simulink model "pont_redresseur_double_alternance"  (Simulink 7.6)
settings: Solver=ode15s  StartTime=0.0  StopTime=0.05  RelTol=1e-3
StopFcn:
  | close all
  | load signaux.mat
  | plot(x(1,:),x(2,:),x(1,:),x(3,:))
  | title('Sinusoide d''entrée et après redressement')
  | grid
  | xlabel('temps')
libraries: fl_lib x13, nesl_utility x3

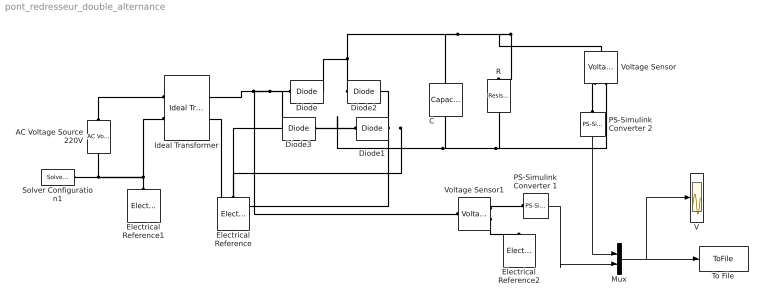
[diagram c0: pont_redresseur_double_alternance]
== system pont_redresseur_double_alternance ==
  AC Voltage Source 220V : fl_lib/Electrical/Electrical Sources/AC Voltage Source  DialogController=NetworkEngine.DynNeDlgSource  SystemSampleTime=-1  amp=220 V  shift=0 rad  omega=60 Hz  i_Log=off  v_Log=off  LocalVarNames=|i|v  LocalVarDescs=|i|v  LocalVarLogging=[0 0]
  C : fl_lib/Electrical/Electrical Elements/Capacitor  DialogController=NetworkEngine.DynNeDlgSource  SystemSampleTime=-1  c=1e-03 F  v0=0 V  r=1e-06 Ohm  g=0 1/Ohm  i_Log=off  v_Log=off  vc_Log=off  LocalVarNames=|i|v|vc  LocalVarDescs=|i|v|Internal variable for voltage across capacitor term  LocalVarLogging=[0 0 0]
  Diode{,1..3} (4 alike) : fl_lib/Electrical/Electrical Elements/Diode  DialogController=NetworkEngine.DynNeDlgSource  SystemSampleTime=-1  Vf=0.6 V  Ron=0.3 Ohm  Goff=1e-08 1/Ohm  i_Log=off  v_Log=off  LocalVarNames=|i|v  LocalVarDescs=|i|v  LocalVarLogging=[0 0]
  Electrical Reference : fl_lib/Electrical/Electrical Elements/Electrical Reference  DialogController=NetworkEngine.DynNeDlgSource  SystemSampleTime=-1  i_Log=off  LocalVarNames=|i  LocalVarDescs=|i  LocalVarLogging=0
  Electrical Reference1 : fl_lib/Electrical/Electrical Elements/Electrical Reference  DialogController=NetworkEngine.DynNeDlgSource  SystemSampleTime=-1  i_Log=off  LocalVarNames=|i  LocalVarDescs=|i  LocalVarLogging=0
  Electrical Reference2 : fl_lib/Electrical/Electrical Elements/Electrical Reference  DialogController=NetworkEngine.DynNeDlgSource  SystemSampleTime=-1  i_Log=off  LocalVarNames=|i  LocalVarDescs=|i  LocalVarLogging=0
  Ideal Transformer : fl_lib/Electrical/Electrical Elements/Ideal Transformer  DialogController=NetworkEngine.DynNeDlgSource  SystemSampleTime=-1  n=18  i1_Log=off  v1_Log=off  i2_Log=off  v2_Log=off  LocalVarNames=|i1|v1|i2|v2  LocalVarDescs=|i1|v1|i2|v2  LocalVarLogging=[0 0 0 0]
  Mux : Mux  Inputs=2
  PS-Simulink Converter 1 : nesl_utility/PS-Simulink Converter  DialogController=NetworkEngine.DynNeUtilDlgSource  SystemSampleTime=-1  PhysicalDomain=network_engine_domain  LeftPortType=input  RightPortType=output  SubClassName=ps_output  Unit=1  AffineConversion=off
  PS-Simulink Converter 2 : nesl_utility/PS-Simulink Converter  DialogController=NetworkEngine.DynNeUtilDlgSource  SystemSampleTime=-1  PhysicalDomain=network_engine_domain  LeftPortType=input  RightPortType=output  SubClassName=ps_output  Unit=1  AffineConversion=off
  R : fl_lib/Electrical/Electrical Elements/Resistor  Tag=Factory Generic  DialogController=NetworkEngine.DynNeDlgSource  SystemSampleTime=-1  R=10e3 Ohm  i_Log=off  v_Log=off  LocalVarNames=|current|voltage|power  LocalVarDescs=|Resistor current (A)|Voltage across resistor (V)|Power (W)  LocalVarLogging=[0 0 0]
  Solver Configuration1 : nesl_utility/Solver Configuration  DialogController=NetworkEngine.DynNeUtilDlgSource  SystemSampleTime=-1  PhysicalDomain=network_engine_domain  LeftPortType=input  RightPortType=generic  SubClassName=solver  Accelerate=off  Profile=off  ResidualTolerance=1e-9  MaxNonlinIter=12  MaxModeIter=2  DoFixedCost=off  UseLocalSampling=off  DoDC=on  LinearAlgebra=Sparse  LocalSolverSampleTime=.001  LocalSolverChoice=NE_BACKWARD_EULER_ADVANCER  UseLocalSolver=off
  To File : ToFile  Filename=signaux  MatrixName=x
  V : Scope
  Voltage Sensor : fl_lib/Electrical/Electrical Sensors/Voltage Sensor  DialogController=NetworkEngine.DynNeDlgSource  SystemSampleTime=-1  i1_Log=off  v1_Log=off  LocalVarNames=|i1|v1  LocalVarDescs=|i1|v1  LocalVarLogging=[]
  Voltage Sensor1 : fl_lib/Electrical/Electrical Sensors/Voltage Sensor  DialogController=NetworkEngine.DynNeDlgSource  SystemSampleTime=-1  i1_Log=off  v1_Log=off  LocalVarNames=|i1|v1  LocalVarDescs=|i1|v1  LocalVarLogging=[]
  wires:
  PS-Simulink Converter 2/1 -> Mux/1
  PS-Simulink Converter 1/1 -> Mux/2
  Mux/1 -> To File/1, V/1
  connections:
  Diode2/RConn1 -- C/LConn1 -- Voltage Sensor/LConn1 -- R/LConn1 -- Diode/RConn1
  PS-Simulink Converter 2/LConn1 -- Voltage Sensor/RConn1
  Diode3/RConn1 -- Diode/LConn1 -- Voltage Sensor1/LConn1 -- Ideal Transformer/RConn1
  Diode2/LConn1 -- Diode1/RConn1 -- Electrical Reference/LConn1 -- Ideal Transformer/RConn2
  Voltage Sensor/RConn2 -- Diode3/LConn1 -- Diode1/LConn1 -- C/RConn1 -- R/RConn1
  AC Voltage Source 220V/RConn1 -- Solver Configuration1/RConn1 -- Electrical Reference1/LConn1 -- Ideal Transformer/LConn2
  Voltage Sensor1/RConn1 -- PS-Simulink Converter 1/LConn1
  Voltage Sensor1/RConn2 -- Electrical Reference2/LConn1
  AC Voltage Source 220V/LConn1 -- Ideal Transformer/LConn1
